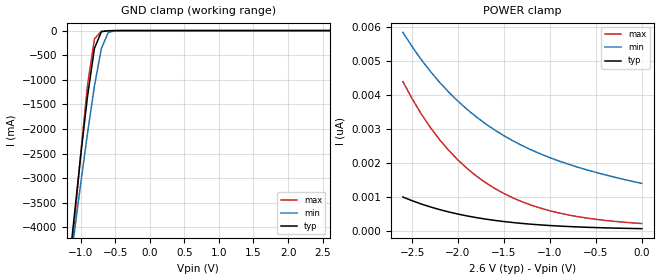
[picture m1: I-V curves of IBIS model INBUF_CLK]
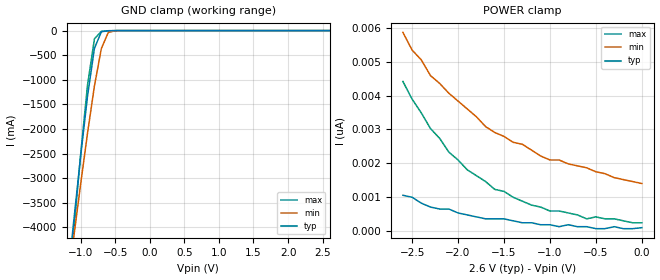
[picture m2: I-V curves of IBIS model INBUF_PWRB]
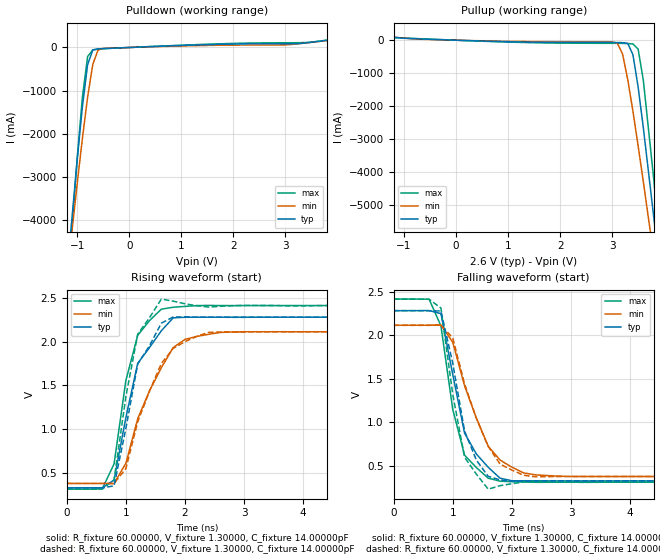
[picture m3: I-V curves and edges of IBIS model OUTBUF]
| IBIS file cspt857_mlf_2p6.ibs created by s2ibis2 version 1.2
| North Carolina State University Electronics Research Laboratory  1995
[IBIS ver]   2.1
[File name]   cspt857c_mlf_2p6.ibs
[File Rev]   1.0
[Date]   Friday, May 09, 2003
[Source]   IDT
[Notes]   1. Temp typ=25C, min=0C, max=100C
   2. IDT's 2.0v C11.5 process
   3. Ramp rate based on 50 ohm load
READ THESE TERMS AND CONDITIONS CAREFULLY BEFORE USING THIS IBIS MODEL.  BY
USING THIS IBIS MODEL, YOU ARE ACCEPTING AND AGREEING TO THESE TERMS AND
CONDITIONS OF USE.
Integrated Device Technology, Inc. ("IDT") hereby grants the user of this
IBIS model ("User") a non-exclusive, nontransferable license to use this
IBIS model under the following terms: The User is granted this license only
to use the IBIS model for demonstration purposes only and is not granted
rights to sell, copy (except as needed to run the IBIS model), rent, lease
or sub-license (except for demonstration) the IBIS model in whole or in
part, or in modified form to anyone. The User may modify the IBIS model to
suit its specific applications, but  rights to derivative works and such
modifications shall belong to IDT.
THIS IBIS MODEL IS PROVIDED ON AN AS IS" BASIS AND IDT  MAKES ABSOLUTELY NO
WARRANTY WITH RESPECT TO THE INFORMATION CONTAINED HEREIN.  IDT DISCLAIMS
AND USER WAIVES ALL WARRANTIES, EXPRESS AND IMPLIED, INCLUDING WARRANTIES OF
MERCHANTABILITY AND FITNESS FOR A PARTICULAR PURPOSE.  THE ENTIRE RISK AS TO
QUALITY AND PERFORMANCE IS WITH THE USER  ACCORDINGLY, IN NO EVENT SHALL IDT
BE LIABLE FOR ANY DIRECT OR INDIRECT DAMAGES, WHETHER IN CONTRACT OR TORT,
INCLUDING ANY LOST PROFITS OR OTHER INCIDENTAL, CONSEQUENTIAL, EXEMPLARY, OR
PUNITIVE DAMAGES ARISING OUT OF THE USE OR APPLICATION OF THE  IBIS MODEL,
WHETHER OR NOT IDT HAD NOTICE OF SUCH DAMAGES.
IDT reserves the right to make changes without notice to any product herein
to improve
reliability, function, or design. IDT does not convey any license under
patent rights or any other intellectual property rights, including those of
third parties. IDT is not obligated
to provide maintenance or support for the licensed IBIS model.
This model is for the 2.5V Phase Locked Loop Differential 1:10 SDRAM Clock
Driver
[Copyright]
Copyright 2002, Integrated Device Technology, Inc. All rights reserved.
|   Component CPST857C
[Component]   CPST857C
[Manufacturer]   Integrated Device Technology Inc.
[Package]
| variable   typ   min   max
R_pkg   86.00000m   61.00000m   0.11300
L_pkg   2.10000nH   1.50000nH   2.70000nH
C_pkg   0.20000pF   0.16000pF   0.24000pF
[Pin]  signal_name   model_name   R_pin   L_pin   C_pin
1   GND   GND
2   _Y2_   OUTBUF
3   Y2   OUTBUF
4   VDDQ   POWER
5   CLK   INBUF_CLK
6   _CLK_   INBUF_CLK
7   VDDQ   POWER
8   AVDD   POWER
9   AGND   GND
10   GND   GND
11   _Y3_   OUTBUF
12   Y3   OUTBUF
13   VDDQ   POWER
14   Y4   OUTBUF
15   _Y4_   OUTBUF
16   _Y9_   OUTBUF
17   Y9   OUTBUF
18   VDDQ   POWER
19   Y8   OUTBUF
20   _Y8_   OUTBUF
21   FBOUT   OUTBUF
22   _FBOUT_   OUTBUF
23   VDDQ   POWER
24   VDDQ   POWER
25   _FBIN_   INBUF_FBIN
26   FBIN   INBUF_FBIN
27   _PWRDWN_   INBUF_PWRB
28   VDDQ   POWER
29   Y7   OUTBUF
30   _Y7_   OUTBUF
31   _Y6_   OUTBUF
32   Y6   OUTBUF
33   VDDQ   POWER
34   Y5   OUTBUF
35   _Y5_   OUTBUF
36   _Y0_   OUTBUF
37   Y0   OUTBUF
38   VDDQ   POWER
39   Y1   OUTBUF
40   _Y1_   OUTBUF
| in   in   dummy_model
[Diff Pin]  inv_pin  vdiff   tdelay_typ  tdelay_min  tdelay_max
5   6   1.00000V  NA  |CLK<P:N> Clock Input  Pair
26   25   1.00000V  NA  |FBIN<P:N> FBIN Input  Pair
3   2   0.000V   NA  |Y2<P:N> Ouput  Pair
12   11   0.000V   NA  |Y3<P:N> Ouput  Pair
14   15   0.000V   NA  |Y4<P:N> Ouput  Pair
17   16   0.000V   NA  |Y9<P:N> Ouput  Pair
19   20   0.000V   NA  |Y8<P:N> Ouput  Pair
21   22   0.000V   NA  |FBOUT<P:N> Ouput  Pair
29   30   0.000V   NA  |Y7<P:N> Ouput  Pair
32   31   0.000V   NA  |Y6<P:N> Ouput  Pair
34   35   0.000V   NA  |Y5<P:N> Ouput  Pair
37   36   0.000V   NA  |Y0<P:N> Ouput  Pair
39   40   0.000V   NA  |Y1<P:N> Ouput  Pair
| Models and submodels in the file (4): INBUF_CLK (Input), INBUF_PWRB (Input), INBUF_FBIN (Input), OUTBUF (Output)
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|   Model INBUF_CLK
[Model]   INBUF_CLK
Model_type   Input
Polarity   Non-Inverting
Vinl =  0.80000V
Vinh =  2.00000V
C_comp   3.50000pF   3.50000pF   3.50000pF
[Temperature Range]   25.00000   100.00000   0.000
[Voltage Range]   2.60000V   2.50000V   2.70000V
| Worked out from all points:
|   GND clamp passes 1 mA (typ) near -0.52 V on its own axis
[GND_clamp]
| voltage   I(typ)   I(min)   I(max)
-2.6V     -25.34A    -21.53A    -29.72A
-1.2V     -5.248A    -5.316A    -5.713A
-1.1V     -3.884A    -4.209A    -4.089A
-1V       -2.564A    -3.127A    -2.526A
-900mV    -1.335A    -2.086A    -1.108A
-800mV    -361.3mA   -1.127A    -168.2mA
-700mV    -23.9mA    -365.3mA   -14.69mA
-600mV    -2.784mA   -39.09mA   -5.291mA
-500mV    -459.2uA   -2.159mA   -1.358mA
2.6V      75.77pA    1.461nA    209.7pA
[POWER_clamp]
| voltage   I(typ)   I(min)   I(max)
-2.6V     1.003nA    5.831nA    4.388nA
-2.5V     895.5pA    5.414nA    3.887nA
-2.4V     798.8pA    5.033nA    3.439nA
-2.3V     712pA      4.684nA    3.039nA
-2.1V     565pA      4.076nA    2.367nA
-1.9V     448.2pA    3.57nA     1.838nA
-1.8V     399.3pA    3.35nA     1.618nA
-1.6V     317.8pA    2.967nA    1.255nA
-1.3V     228.2pA    2.509nA    861.2pA
-900mV    152.1pA    2.058nA    534.7pA
-500mV    107.5pA    1.726nA    349.9pA
0V        75.77pA    1.402nA    226.3pA
|   Model INBUF_PWRB
[Model]   INBUF_PWRB
Model_type   Input
Polarity   Non-Inverting
Vinl =  0.80000V
Vinh =  2.00000V
C_comp   3.50000pF   3.50000pF   3.50000pF
[Temperature Range]   25.00000   100.00000   0.000
[Voltage Range]   2.60000V   2.50000V   2.70000V
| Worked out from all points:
|   GND clamp passes 1 mA (typ) near -0.52 V on its own axis
[GND_clamp]
| voltage   I(typ)   I(min)   I(max)
-2.6V     -25.34A    -21.53A    -29.72A
-1.2V     -5.247A    -5.316A    -5.712A
-1.1V     -3.884A    -4.209A    -4.088A
-1V       -2.564A    -3.127A    -2.526A
-900mV    -1.335A    -2.086A    -1.108A
-800mV    -361.3mA   -1.126A    -168.2mA
-700mV    -23.9mA    -365.3mA   -14.69mA
-600mV    -2.784mA   -39.09mA   -5.291mA
-500mV    -459.2uA   -2.159mA   -1.358mA
2.6V      87.31pA    1.455nA    232.8pA
[POWER_clamp]
| voltage   I(typ)   I(min)   I(max)
-2.6V     1.048nA    5.879nA    4.424nA
-2.5V     989.5pA    5.355nA    3.9nA
-2.4V     814.9pA    5.064nA    3.492nA
-2.3V     698.5pA    4.598nA    3.027nA
-2.2V     640.3pA    4.366nA    2.736nA
-2.1V     640.3pA    4.075nA    2.328nA
-1.9V     465.7pA    3.609nA    1.804nA
-1.6V     349.2pA    2.91nA     1.222nA
-1V       174.6pA    2.095nA    582.1pA
-600mV    116.4pA    1.863nA    349.2pA
-500mV    58.21pA    1.746nA    407.5pA
0V        87.31pA    1.397nA    232.8pA
|   Model OUTBUF
[Model]   OUTBUF
Model_type   Output
Polarity   Non-Inverting
Vmeas =  1.30000V
C_comp   3.50000pF   3.50000pF   3.50000pF
[Temperature Range]   25.00000   100.00000   0.000
[Voltage Range]   2.60000V   2.50000V   2.70000V
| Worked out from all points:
|   slope of the pulldown table from 0 to 0.39 V, typ, clamps not added: 20.1 ohm
|   slope of the pullup table from 0 to 0.39 V, typ, clamps not added: 19.5 ohm
|   rising waveform, R_fixture 60.00000, V_fixture 1.30000, C_fixture 14.00000pF: 20-80 % time 468ps typ, 610ps min, 341ps max; typ from 0.326 V to 2.28 V
|   rising waveform, R_fixture 60.00000, V_fixture 1.30000, C_fixture 14.00000pF: 20-80 % time 426ps typ, 551ps min, 308ps max; typ from 0.326 V to 2.28 V
|   falling waveform, R_fixture 60.00000, V_fixture 1.30000, C_fixture 14.00000pF: 20-80 % time 429ps typ, 539ps min, 335ps max; typ from 2.28 V to 0.326 V
|   falling waveform, R_fixture 60.00000, V_fixture 1.30000, C_fixture 14.00000pF: 20-80 % time 379ps typ, 522ps min, 299ps max; typ from 2.28 V to 0.326 V
[Pulldown]
| voltage   I(typ)   I(min)   I(max)
-2.6V     -25.48A    -21.66A    -29.86A
-1.2V     -5.305A    -5.362A    -5.777A
-1V       -2.612A    -3.165A    -2.58A
-900mV    -1.379A    -2.12A     -1.157A
-800mV    -400.6mA   -1.157A    -211.8mA
-700mV    -58.58mA   -392.6mA   -53.12mA
-600mV    -32.75mA   -62.73mA   -38.49mA
-500mV    -25.6mA    -22.07mA   -29.24mA
1.8V      74.65mA    53.14mA    87.89mA
3V        87.07mA    61.25mA    109.7mA
3.3V      95.16mA    92.97mA    112.3mA
5.2V      400.4mA    370.7mA    414.1mA
[Pullup]
| voltage   I(typ)   I(min)   I(max)
-2.6V     302.8mA    288.1mA    310.8mA
-900mV    51.47mA    51.29mA    59.76mA
1.3V      -54.7mA    -38.46mA   -68.74mA
3.1V      -70.01mA   -89.45mA   -94.24mA
3.2V      -73.17mA   -420.6mA   -95.98mA
3.3V      -96.9mA    -1.187A    -101.2mA
3.4V      -439.3mA   -2.153A    -112.7mA
3.5V      -1.419A    -3.2A      -270mA
3.6V      -2.655A    -4.288A    -1.216A
3.8V      -5.352A    -6.531A    -4.21A
4V        -8.161A    -8.821A    -7.507A
5.2V      -25.55A    -22.89A    -28.21A
[Ramp]
| variable   typ   min   max
dV/dt_r   1.09920/0.10519n   0.93300/0.15232n   1.21080/0.13672n
dV/dt_f   1.10088/0.14109n   0.96540/0.13417n   1.18398/0.13634n
R_load = 50.00000
[Rising Waveform]
R_fixture = 60.00000
V_fixture = 1.30000
V_fixture_min = 1.25000
V_fixture_max = 1.35000
C_fixture = 14.00000pF
| time   V(typ)   V(min)   V(max)
0s        325.5mV    375.9mV    310.2mV
600ps     325.4mV    375.9mV    313.6mV
800ps     415.9mV    374.8mV    599.6mV
1ns       1.132V     607mV      1.557V
1.2ns     1.754V     1.119V     2.076V
1.6ns     2.128V     1.704V     2.376V
1.8ns     2.276V     1.935V     2.397V
2ns       2.283V     2.029V     2.408V
2.6ns     2.284V     2.109V     2.417V
10ns      2.284V     2.116V     2.417V
[Rising Waveform]
R_fixture = 60.00000
V_fixture = 1.30000
V_fixture_min = 1.25000
V_fixture_max = 1.35000
C_fixture = 14.00000pF
R_dut = 86.00000m
L_dut = 2.10000nH
C_dut = 0.20000pF
| time   V(typ)   V(min)   V(max)
0s        326.5mV    376.8mV    311.4mV
600ps     326.5mV    376.8mV    311.4mV
800ps     347.7mV    376.1mV    416.1mV
1ns       1.008V     546.7mV    1.374V
1.2ns     1.746V     1.082V     2.088V
1.4ns     1.957V     1.435V     2.279V
1.6ns     2.215V     1.752V     2.491V
1.8ns     2.285V     1.925V     2.467V
2.4ns     2.284V     2.11V      2.4V
10ns      2.283V     2.115V     2.415V
[Falling Waveform]
R_fixture = 60.00000
V_fixture = 1.30000
V_fixture_min = 1.25000
V_fixture_max = 1.35000
C_fixture = 14.00000pF
| time   V(typ)   V(min)   V(max)
0s        2.284V     2.116V     2.417V
600ps     2.285V     2.116V     2.415V
800ps     2.25V      2.12V      2.108V
1ns       1.547V     1.92V      1.147V
1.2ns     874.7mV    1.418V     621.2mV
1.4ns     634.4mV    1.047V     478.8mV
1.6ns     482.4mV    723.4mV    356.9mV
1.8ns     356.9mV    565.6mV    322.2mV
2.4ns     326mV      395.1mV    309.7mV
10ns      325.5mV    375.9mV    310.2mV
[Falling Waveform]
R_fixture = 60.00000
V_fixture = 1.30000
V_fixture_min = 1.25000
V_fixture_max = 1.35000
C_fixture = 14.00000pF
R_dut = 86.00000m
L_dut = 2.10000nH
C_dut = 0.20000pF
| time   V(typ)   V(min)   V(max)
0s        2.283V     2.115V     2.415V
600ps     2.283V     2.115V     2.415V
800ps     2.28V      2.117V     2.313V
1ns       1.677V     1.97V      1.319V
1.2ns     899.1mV    1.441V     597.9mV
1.4ns     563.5mV    1.042V     402.2mV
1.6ns     377.7mV    721.9mV    230.6mV
1.8ns     336.4mV    519.3mV    270.9mV
2.4ns     325.2mV    372.3mV    320.4mV
10ns      326.5mV    376.8mV    311.4mV
